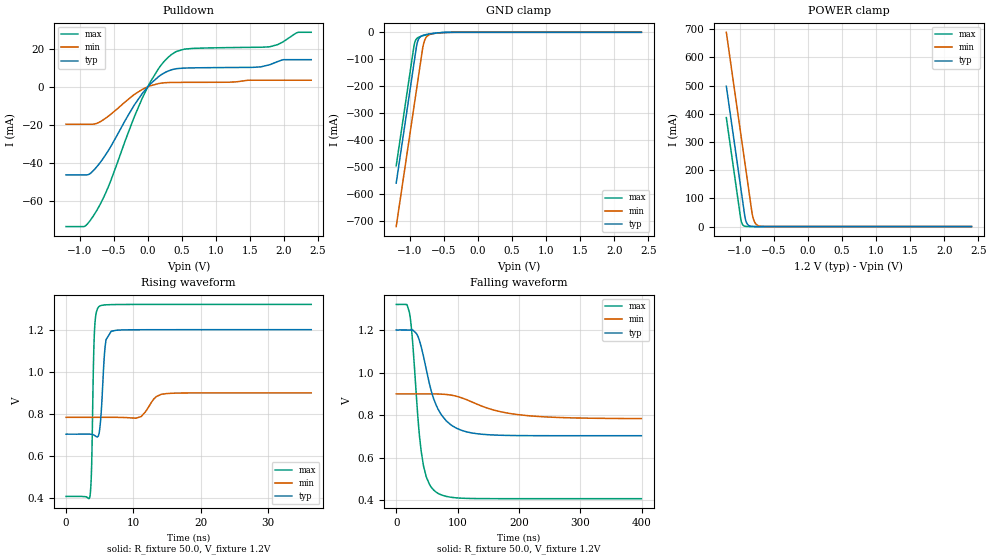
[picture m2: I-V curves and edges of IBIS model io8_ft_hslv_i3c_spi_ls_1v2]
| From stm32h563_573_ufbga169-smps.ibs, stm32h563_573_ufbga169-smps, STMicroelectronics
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[Model]   io8_ft_hslv_i3c_spi_ls_1v2
Model_type I/O_open_drain
Polarity   Non-Inverting
Enable   Active-Low
| CAP_THRESHOLD on pad IOFT is "UDTCAPC" :
| Rising=20.0% of vddiom   Falling=80.0% of vddiom
| C_comp min and max val. don't necessarily correlate with the min and max pvt
| but are the smallest and greatest pad capacitance found.
| var   typ   min   max
C_comp   3.41625pF  3.40150pF  3.42905pF
|C_comp_pulldown   3.41625pF  3.40150pF  3.42905pF
Vinl = 450.0mV
Vinh = 660.0mV
Vmeas = 600.0mV   | Reference voltage for timing measurements
Cref  = 50.0pF   | Timing specification test load capacitance value
Rref  = 1.0MOhm   | Timing specification test load resistance value
Vref  = 660.0mV   | Timing specification test load voltage
[Model Spec]
| TIME_THRESHOLD on pin ZII2CV11 is "CMOS" :
| Rising=40.0% of vdd   Falling=60.0% of vdd
Vinl 447.80000mV 344.80000mV 489.80000mV
Vinh 733.20000mV 535.20000mV 813.20000mV
| variable   typ   min   max
[Temperature Range] 25.0 125.0 -40.0
| variable   typ   min   max
[Voltage Range] 1.2V 900.0mV 1.32V
| variable   typ   min   max
[POWER Clamp Reference] 1.2V 900.0mV 1.32V
| variable   typ   min   max
[GND Clamp Reference] 0V 0V 0V
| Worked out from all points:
|   slope of the pulldown table from 0 to 0.18 V, typ, clamps not added: 30.6 ohm
|   GND clamp passes 1 mA (typ) near -0.52 V on its own axis
|   POWER clamp passes 1 mA (typ) near -0.84 V on its own axis
|   rising waveform, R_fixture 50.0, V_fixture 1.2V: 20-80 % time 539ps typ, 1.52ns min, 327ps max; typ from 0.704 V to 1.2 V
|   falling waveform, R_fixture 50.0, V_fixture 1.2V: 20-80 % time 30.8ns typ, 76.2ns min, 16ns max; typ from 1.2 V to 0.704 V
[POWER Clamp]
-1.2V     497.8mA    689.2mA    386.5mA
-990mV    140.8mA    332.2mA    29.53mA
-980mV    123.8mA    315.2mA    17.95mA
-960mV    89.81mA    281.2mA    6.634mA
-930mV    38.81mA    230.2mA    1.49mA
-900mV    12.07mA    179.2mA    334.8uA
-870mV    3.756mA    128.2mA    75.22uA
-820mV    536.4uA    44.98mA    6.246uA
-790mV    166.9uA    18.76mA    1.403uA
-750mV    35.18uA    5.846mA    191.8nA
-590mV    70.09nA    55uA       165.5pA
2.4V      0A         0A         0A
[GND Clamp]
-1.2V     -558.2mA   -719mA     -494.1mA
-940mV    -116.2mA   -277mA     -52.06mA
-930mV    -99.19mA   -260mA     -39.94mA
-900mV    -49.1mA    -209mA     -23.76mA
-880mV    -30.14mA   -175mA     -19.6mA
-850mV    -17.82mA   -124mA     -16.09mA
-810mV    -11.73mA   -56.78mA   -12.91mA
-780mV    -9.444mA   -28.21mA   -10.92mA
-740mV    -7.291mA   -13.16mA   -8.574mA
-640mV    -3.573mA   -4.171mA   -3.954mA
-380mV    -61.75uA   -230.3uA   -20.32uA
2.4V      3.863nA    718.4nA    150.6pA
| variable   typ   min   max
[Pullup Reference] 1.2V 900.0mV 1.32V
| variable   typ   min   max
[Pulldown Reference] 0V 0V 0V
[Pulldown]
-1.2V     -46.17mA   -19.62mA   -73.27mA
-930mV    -46.17mA   -19.62mA   -73.18mA
-770mV    -42.8mA    -19.4mA    -66.04mA
-570mV    -32.88mA   -15.18mA   -51.58mA
-80mV     -3.488mA   -1.363mA   -5.887mA
160mV     5.368mA    1.685mA    9.621mA
340mV     8.782mA    2.25mA     16.66mA
540mV     9.805mA    2.305mA    19.74mA
1.79V     11.53mA    3.427mA    20.94mA
1.98V     14.11mA    3.427mA    23.43mA
2.2V      14.2mA     3.427mA    28.44mA
2.4V      14.2mA     3.427mA    28.54mA
[Ramp]
dV/dt_r 297.78132mV/539.24904ps 69.85344mV/1.48528ns 547.12198mV/325.15187ps
dV/dt_f 297.8048mV/30.76971ns 69.58345mV/75.96303ns 547.1393mV/15.8192ns
R_load = 50.0
| Removed startup time: 0s 0s 0s  .
| Removed end time: 36.4ns.
[Rising Waveform]
R_fixture   = 50.0
V_fixture   = 1.2V
V_fixture_min = 900.0mV
V_fixture_max = 1.32V
0s        703.7mV    783.5mV    408.1mV
3.55ns    703.7mV    783.5mV    410.3mV
3.8ns     703.1mV    783.5mV    560.6mV
4.05ns    700.7mV    783.5mV    1.014V
4.2ns     698.2mV    783.5mV    1.182V
4.9ns     708.1mV    783.5mV    1.31V
5.85ns    1.133V     783.5mV    1.318V
6.7ns     1.192V     783.5mV    1.319V
14.9ns    1.2V       896.3mV    1.32V
36.4ns    1.2V       899.9mV    1.32V
| Removed startup time: 0s 0s 0s  .
| Removed end time: 399.4ns.
[Falling Waveform]
R_fixture   = 50.0
V_fixture   = 1.2V
V_fixture_min = 900.0mV
V_fixture_max = 1.32V
0s        1.2V       900mV      1.32V
21.25ns   1.2V       900mV      1.285V
25.7ns    1.2V       900mV      1.18V
35.65ns   1.168V     900mV      777.8mV
40.75ns   1.121V     900mV      629.7mV
48.9ns    1.016V     900mV      511.3mV
65.2ns    846.4mV    899.8mV    438.5mV
89.65ns   753.3mV    894.4mV    414.5mV
130.5ns   713.5mV    853.3mV    408.6mV
399.4ns   703.7mV    784mV      408.1mV
